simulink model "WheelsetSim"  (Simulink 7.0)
settings: Solver=ode45  StartTime=0.0  StopTime=20  RelTol=1e-3
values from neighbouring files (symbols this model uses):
  K = [-1 -3 -3 0 0 0    [init.m]
libraries: simulink x1

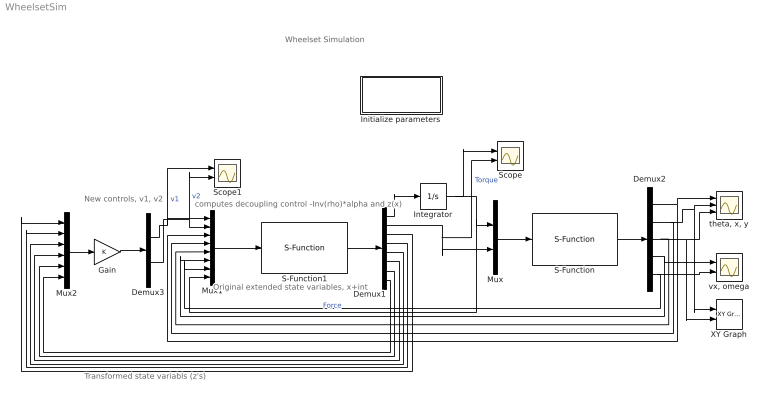
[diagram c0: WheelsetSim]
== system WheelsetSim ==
  note: Wheelset Simulation
  note: Original extended state variables, x+int
  note: Transformed state variabls (z's)
  note: New controls, v1, v2
  note: computes decoupling control -Inv(rho)*alpha and z(x)
  Demux1 : Demux  Outputs=8
  Demux2 : Demux  Outputs=5
  Demux3 : Demux  Outputs=2
  Gain : Gain  Gain=K  Multiplication=Matrix(K*u) (u vector)  ParameterDataType=sfix(16)  ParameterScaling=2^0  OutDataType=sfix(16)  OutScaling=2^0
  Initialize parameters : Subsystem
  Integrator : Integrator
  Mux : Mux  Inputs=2
  Mux1 : Mux  Inputs=8
  Mux2 : Mux  Inputs=6
  S-Function : S-Function  FunctionName=wheelset  Parameters=[pi/4;0;0;10;0];[1];[1]
  S-Function1 : S-Function  FunctionName=decoupling  Parameters=[]
  Scope : Scope  NumInputPorts=2
  Scope1 : Scope  NumInputPorts=2
  XY Graph : simulink/Sinks/XY Graph  SystemSampleTime=-1  xmin=-1  xmax=10  ymin=-1  ymax=10  st=-1
  "theta, x, y" : Scope  NumInputPorts=3
  "vx, omega" : Scope  NumInputPorts=2
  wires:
  Demux2/1 -> "theta, x, y"/1, Mux1/3
  Demux2/2 -> Mux1/4, "theta, x, y"/2, XY Graph/1
  Demux2/3 -> Mux1/5, "theta, x, y"/3, XY Graph/2
  Demux2/4 -> "vx, omega"/1, Mux1/6
  Demux2/5 -> "vx, omega"/2, Mux1/7
  ? -> ?
  Integrator/1 -> Mux/1, Mux1/8, Scope/1  "Force"
  Mux1/1 -> S-Function1/1
  S-Function1/1 -> Demux1/1
  Demux1/1 -> Integrator/1
  Mux/1 -> S-Function/1
  S-Function/1 -> Demux2/1
  Mux2/1 -> Gain/1
  Gain/1 -> Demux3/1
  Demux1/2 -> Mux/2, Scope/2  "Torque"
  Demux3/1 -> Mux1/1, Scope1/1  "v1"
  Demux3/2 -> Mux1/2, Scope1/2  "v2"
  Demux1/8 -> Mux2/6
  Demux1/7 -> Mux2/5
  Demux1/6 -> Mux2/4
  Demux1/5 -> Mux2/3
  Demux1/4 -> Mux2/2
  Demux1/3 -> Mux2/1

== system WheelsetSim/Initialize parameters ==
  note: Masked block has FcnOpen Callback associated with init.m to declare SAS parameters
